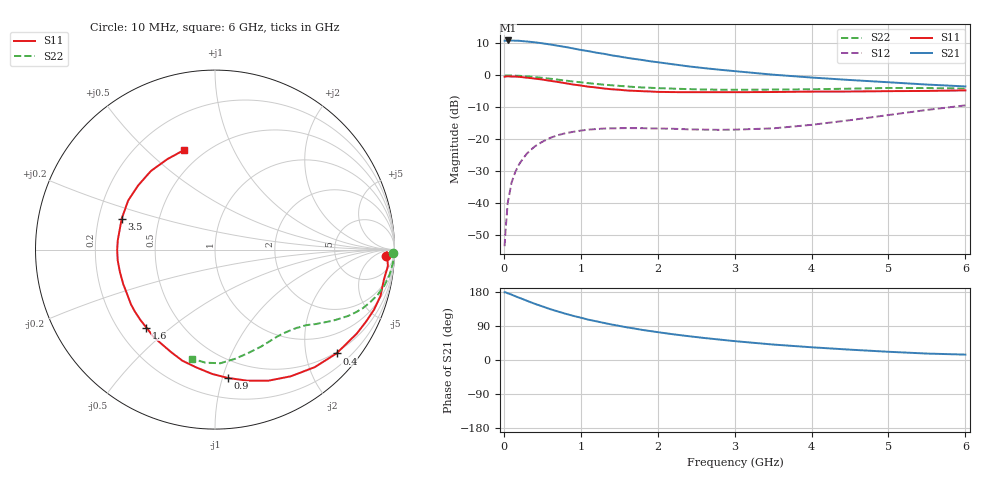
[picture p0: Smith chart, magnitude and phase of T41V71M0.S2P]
! Infineon Technologies  Discrete & RF Semiconductors
! BFR182T
! Si NPN RF Bipolar Junction Transistor in SC75
! VCE = 1.75 V  IC = 1 mA
! Common Emitter S-Parameters:  October  1999
# GHz  S  MA  R  50
!  f  S11  S21  S12  S22
! GHz  MAG  ANG  MAG  ANG  MAG  ANG  MAG  ANG
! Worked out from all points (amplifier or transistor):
!   36 points, 10 MHz to 6 GHz, reference 50 ohm
!   highest |S21| = 10.9 dB at 50 MHz (marker M1)
!   |S21| within 3 dB of that: start of sweep to 1.009 GHz
!   unconditionally stable (mu >= 1): 2.359 GHz to 4.636 GHz
!   at 250 MHz: K = 0.09, MSG = 18.4 dB, |S12| = -26.1 dB
!   at 1.4 GHz: K = 0.59, MSG = 11.4 dB, |S12| = -16.6 dB
!   at 6 GHz: K = 0.86, MSG = 3.0 dB, |S12| = -9.4 dB
!   S11 on the Smith chart (normalised r, x): 10 MHz: 26, -20; 400 MHz: 0.47, -2.64; 900 MHz: 0.35, -1.04; 1.6 GHz: 0.32, -0.41; 3.5 GHz: 0.30, +0.15; 6 GHz: 0.39, +0.66
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0.01  0.9529 -2.1  3.492 178.7  0.0021 87.4  0.9919 -1.2
0.02  0.9576 -0.8  3.492 178.9  0.0034 94.0  0.9891 -0.8
0.05  0.9677 -5.4  3.522 176.1  0.0099 89.5  0.9972 -2.1
0.1  0.956 -10.0  3.505 172.5  0.0208 85.6  0.9944 -4.1
0.15  0.9575 -15.7  3.497 168.2  0.0308 81.1  0.9883 -6.1
0.25  0.9329 -25.3  3.433 160.4  0.0498 75.2  0.9736 -10.0
0.4  0.8906 -40.5  3.299 148.5  0.0766 66.4  0.9409 -15.5
0.5  0.8589 -49.7  3.178 141.5  0.0909 61.6  0.9142 -18.6
0.6  0.8226 -59.1  3.051 134.4  0.1043 56.6  0.8861 -21.6
0.8  0.753 -76.0  2.783 122.2  0.1237 48.4  0.8285 -26.5
0.9  0.7183 -84.4  2.642 116.6  0.1301 45.3  0.8002 -28.5
1.1  0.664 -99.2  2.393 106.4  0.141 39.6  0.7539 -32.0
1.3  0.6223 -112.9  2.177 97.9  0.1466 35.1  0.714 -35.0
1.4  0.605 -119.1  2.06 93.7  0.1476 33.3  0.699 -36.4
1.6  0.5787 -131.4  1.882 86.2  0.1491 30.6  0.6699 -38.7
1.8  0.5643 -142.2  1.74 79.4  0.1485 29.0  0.6461 -41.4
2.2  0.5461 -159.5  1.49 67.9  0.1454 28.6  0.619 -46.1
2.8  0.5451 -179.7  1.226 54.0  0.1399 33.2  0.5955 -54.5
3.5  0.5477 161.7  1.024 40.8  0.1475 44.3  0.5978 -64.2
4.5  0.5578 140.1  0.845 27.3  0.1982 56.7  0.6184 -79.4
5.5  0.5697 117.8  0.717 17.0  0.2869 58.4  0.6323 -94.8
6  0.5808 107.3  0.67 14.2  0.3383 55.6  0.6209 -102.1
